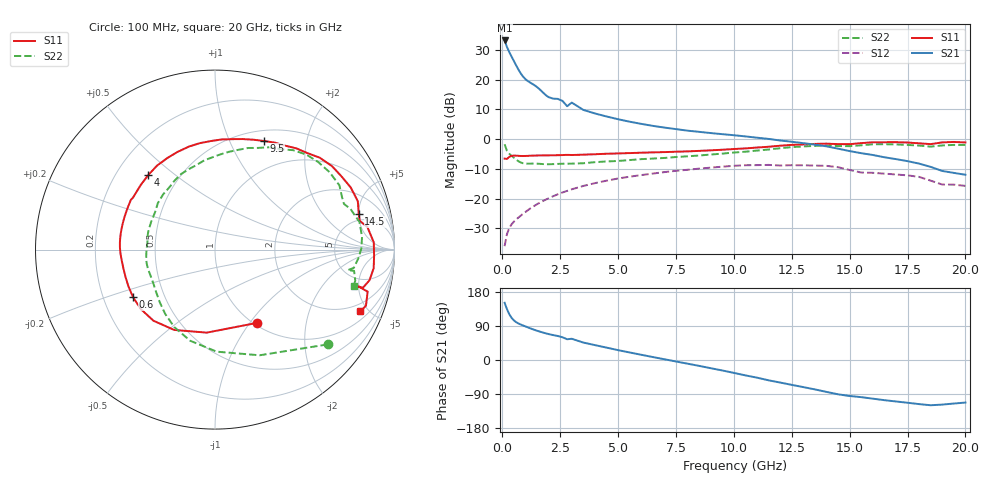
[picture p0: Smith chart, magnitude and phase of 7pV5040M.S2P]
! Infineon Technologies  Discrete & RF Semiconductors
! bfp620
! VCE = 0.50 V,  IC =  40 mA
! Common Emitter S-Parameters:  Sep 2002
# GHz  S  MA  R  50
!  f  S11  S21  S12  S22
! GHz  MAG  ANG  MAG  ANG  MAG  ANG  MAG  ANG
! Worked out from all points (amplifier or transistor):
!   59 points, 100 MHz to 20 GHz, reference 50 ohm
!   highest |S21| = 33.2 dB at 100 MHz (marker M1)
!   |S21| within 3 dB of that: start of sweep to 247.7 MHz
!   unconditionally stable (mu >= 1): 1.937 GHz to 2.268 GHz; 3.128 GHz to 10.3 GHz; 17.04 GHz to end of sweep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
!   at 1 GHz: K = 0.87, MSG = 22.3 dB, |S12| = -24.5 dB
!   at 5.5 GHz: K = 1.06, MAG = 7.8 dB, |S12| = -12.6 dB
!   at 20 GHz: K = 1.70, MAG = -3.0 dB, |S12| = -15.7 dB
!   S11 on the Smith chart (normalised r, x): 100 MHz: 1.03, -1.08; 600 MHz: 0.33, -0.24; 4 GHz: 0.34, +0.40; 9.5 GHz: 0.62, +1.35; 14.5 GHz: 4.05, +5.02; 20 GHz: 1.46, -4.46
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0.1  0.4706 -60.2  45.56 151.0  0.0159 62.1  0.8201 -40.1
0.2  0.4649 -95.7  35.41 134.4  0.0253 53.7  0.6392 -67.1
0.3  0.5022 -117.0  29.12 121.0  0.032 50.9  0.5686 -89.1
0.4  0.5241 -130.9  24.45 111.3  0.037 49.7  0.5262 -105.3
0.5  0.5299 -141.4  20.57 104.5  0.041 49.4  0.4878 -117.7
0.6  0.5278 -150.0  17.31 99.8  0.0447 49.6  0.4527 -127.9
0.8  0.5214 -162.8  12.68 93.5  0.0519 50.5  0.405 -143.9
1  0.5218 -171.1  10.2 88.6  0.0597 51.4  0.3886 -154.8
1.4  0.5301 178.3  8.009 79.3  0.0764 51.8  0.3883 -168.2
1.8  0.5331 168.1  5.86 71.7  0.0931 50.3  0.3805 179.0
2.6  0.5402 153.8  4.392 60.0  0.127 45.0  0.3859 163.2
2.8  0.5446 149.4  3.575 54.8  0.135 43.3  0.3869 157.6
3  0.541 147.6  4.115 56.0  0.1436 41.5  0.3879 157.2
3.5  0.5485 139.0  3.1 46.0  0.1636 36.7  0.3935 148.1
4  0.5575 131.9  2.703 39.3  0.1821 31.8  0.4103 140.9
7  0.6056 91.9  1.565 2.0  0.2793 1.4  0.4827 102.2
9.5  0.6636 65.8  1.213 -27.6  0.3444 -25.5  0.5711 76.8
10.5  0.6985 56.0  1.112 -40.6  0.3644 -38.3  0.615 67.1
13.5  0.8318 24.6  0.809 -77.6  0.3597 -73.8  0.7706 34.0
14.5  0.8251 13.9  0.692 -90.5  0.3375 -89.2  0.7655 22.4
17  0.8902 -6.7  0.462 -109.4  0.2547 -104.9  0.8152 0.4
20  0.8802 -23.0  0.252 -112.3  0.1639 -116.4  0.7986 -14.8
